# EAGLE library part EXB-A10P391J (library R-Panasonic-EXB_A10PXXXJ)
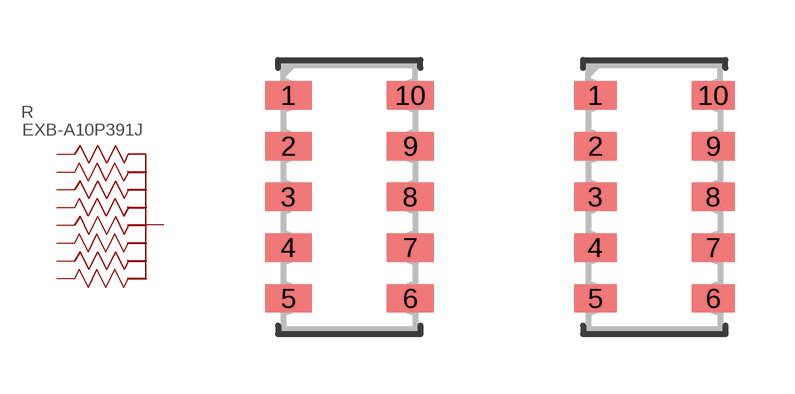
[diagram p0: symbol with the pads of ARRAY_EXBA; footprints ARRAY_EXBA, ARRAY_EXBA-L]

Designator prefix R

## EXB-A10P391J (MANUFACTURER_PART_NUMBER: EXBA10P391J; VENDOR: Panasonic)  [ARRAY_EXBA]
1  11  pas
2  22  pas
3  33  pas
4  44  pas
5  55  pas
6  66  pas
7  77  pas
8  88  pas
9  99  pas
10  55  pas

## EXB-A10P391JC_ARRAY_EXBA-L (MANUFACTURER_PART_NUMBER: EXBA10P391J; VENDOR: Panasonic)  [ARRAY_EXBA-L]
Pads as for ARRAY_EXBA

## EXB-A10P391JC_ARRAY_EXBA-M (MANUFACTURER_PART_NUMBER: EXBA10P391J; VENDOR: Panasonic)  [ARRAY_EXBA-M]
Pads as for ARRAY_EXBA

## Footprint ARRAY_EXBA (pad centres in mm)
smd 1.168 x 0.711: 1 -1.524,2.54; 2 -1.524,1.27; 3 -1.524,0; 4 -1.524,-1.27; 5 -1.524,-2.54; 6 1.524,-2.54; 7 1.524,-1.27; 8 1.524,0; 9 1.524,1.27; 10 1.524,2.54

## Footprint ARRAY_EXBA-L (pad centres in mm)
smd 1.067 x 0.711: 1 -1.473,2.54; 2 -1.473,1.27; 3 -1.473,0; 4 -1.473,-1.27; 5 -1.473,-2.54; 6 1.473,-2.54; 7 1.473,-1.27; 8 1.473,0; 9 1.473,1.27; 10 1.473,2.54

## Footprint ARRAY_EXBA-M (pad centres in mm)
smd 1.27 x 0.711: 1 -1.575,2.54; 2 -1.575,1.27; 3 -1.575,0; 4 -1.575,-1.27; 5 -1.575,-2.54; 6 1.575,-2.54; 7 1.575,-1.27; 8 1.575,0; 9 1.575,1.27; 10 1.575,2.54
